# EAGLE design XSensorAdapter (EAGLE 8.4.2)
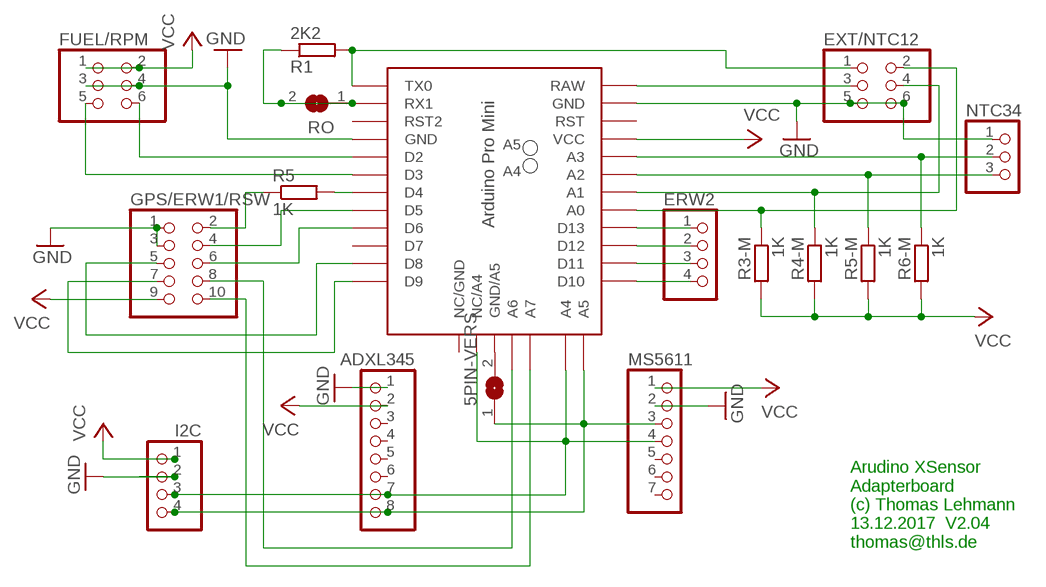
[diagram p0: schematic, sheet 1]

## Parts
5PIN-VERS  SJ  [SJ]
ADXL345  PINHD-1X8  [1X08]
ERW2  PINHD-1X4  [1X04]
EXT/NTC12  PINHD-2X3  [2X03]
FUEL/RPM  PINHD-2X3  [2X03]
GPS/ERW1/RSW  PINHD-2X5  [2X05]
I2C  PINHD-1X4  [1X04]
MS5611  PINHD-1X7  [1X07]
NTC34  PINHD-1X3  [1X03]
R1  2K2  R-EU_0207/10  [0207/10]
R3-M  1K  R-EU_0207/10  [0207/10]
R4-M  1K  R-EU_0207/10  [0207/10]
R5  1K  R-EU_0207/10  [0207/10]
R5-M  1K  R-EU_0207/10  [0207/10]
R6-M  1K  R-EU_0207/10  [0207/10]
RO  SJ  [SJ]
U$1  PRO-MINI-5PINPRO-MINI-5PIN  [PRO-MINI-5PIN]

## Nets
GND: ADXL345.1 EXT/NTC12.5 EXT/NTC12.6 FUEL/RPM.3 FUEL/RPM.4 GPS/ERW1/RSW.1 GPS/ERW1/RSW.3 I2C.2 MS5611.2 NTC34.1 U$1.GND U$1.GND1(GND)
N$1: NTC34.2 R6-M.1 U$1.A3
N$2: EXT/NTC12.1 R1.2 U$1.TX0
N$3: GPS/ERW1/RSW.7 U$1.D9
N$4: EXT/NTC12.3 U$1.RAW
N$5: GPS/ERW1/RSW.10 U$1.A7
N$6: GPS/ERW1/RSW.4 U$1.D5
N$7: GPS/ERW1/RSW.5 U$1.D8
N$8: GPS/ERW1/RSW.6 U$1.D6
N$9: 5PIN-VERS.2 U$1.GND/A5
N$10: EXT/NTC12.2 R3-M.1 U$1.A0
N$11: FUEL/RPM.6 U$1.D2
N$12: R5.2 U$1.D4
N$13: ADXL345.7 I2C.3 MS5611.4 U$1.A5(A4) U$1.NC/A4
N$14: FUEL/RPM.5 U$1.D3
N$15: GPS/ERW1/RSW.2 R5.1
N$16: 5PIN-VERS.1 ADXL345.8 I2C.4 MS5611.3 U$1.A4(A5)
N$17: R1.1 RO.1 RO.2 U$1.RX1
N$18: GPS/ERW1/RSW.8 U$1.A6
N$19: EXT/NTC12.4 R4-M.1 U$1.A1
N$20: NTC34.3 R5-M.1 U$1.A2
N$21: ERW2.1 U$1.D13
N$22: ERW2.2 U$1.D12
N$23: ERW2.3 U$1.D11
N$24: ERW2.4 U$1.D10
VCC: ADXL345.2 FUEL/RPM.1 FUEL/RPM.2 GPS/ERW1/RSW.9 I2C.1 MS5611.1 R3-M.2 R4-M.2 R5-M.2 R6-M.2 U$1.VCC
Unconnected: ADXL345.3 ADXL345.4 ADXL345.5 ADXL345.6 MS5611.5 MS5611.6 MS5611.7 U$1.D7 U$1.NC/GND U$1.RST U$1.RST1(RST2)

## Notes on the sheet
- Arudino XSensor
  Adapterboard
  (c) Thomas Lehmann
  13.12.2017  V2.04
  thomas@thls.de

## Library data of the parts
5PIN-VERS RO = jumper:SJ: SMD solder JUMPER
ADXL345 = pinhead:PINHD-1X8: PIN HEADER
ERW2 I2C = pinhead:PINHD-1X4: PIN HEADER
EXT/NTC12 FUEL/RPM = pinhead:PINHD-2X3: PIN HEADER
GPS/ERW1/RSW = pinhead:PINHD-2X5: PIN HEADER
MS5611 = pinhead:PINHD-1X7: PIN HEADER
NTC34 = pinhead:PINHD-1X3: PIN HEADER
R1 R3-M R4-M R5 R5-M R6-M = resistor:R-EU_: RESISTOR, European symbol
U$1 = OwnLib:PRO-MINI-5PIN

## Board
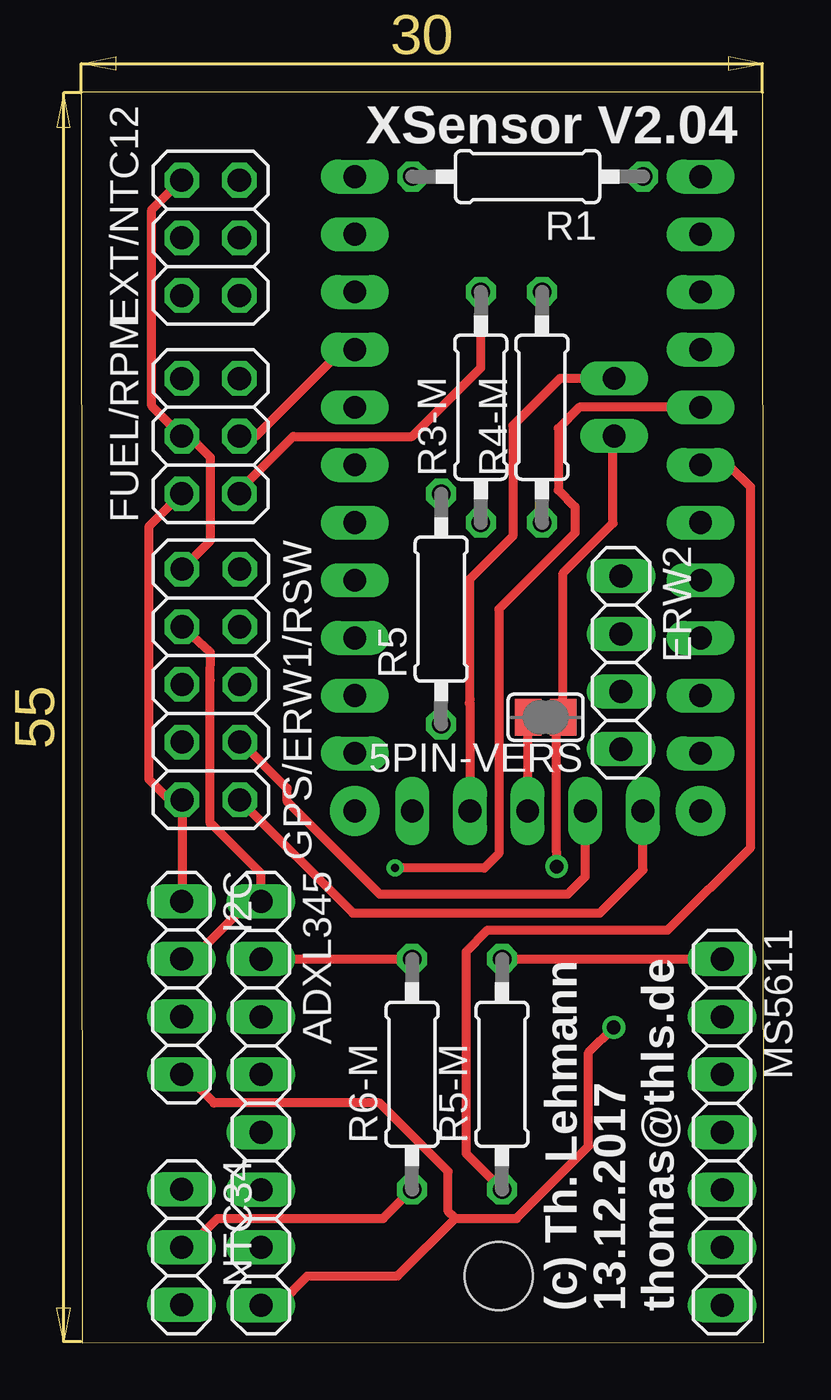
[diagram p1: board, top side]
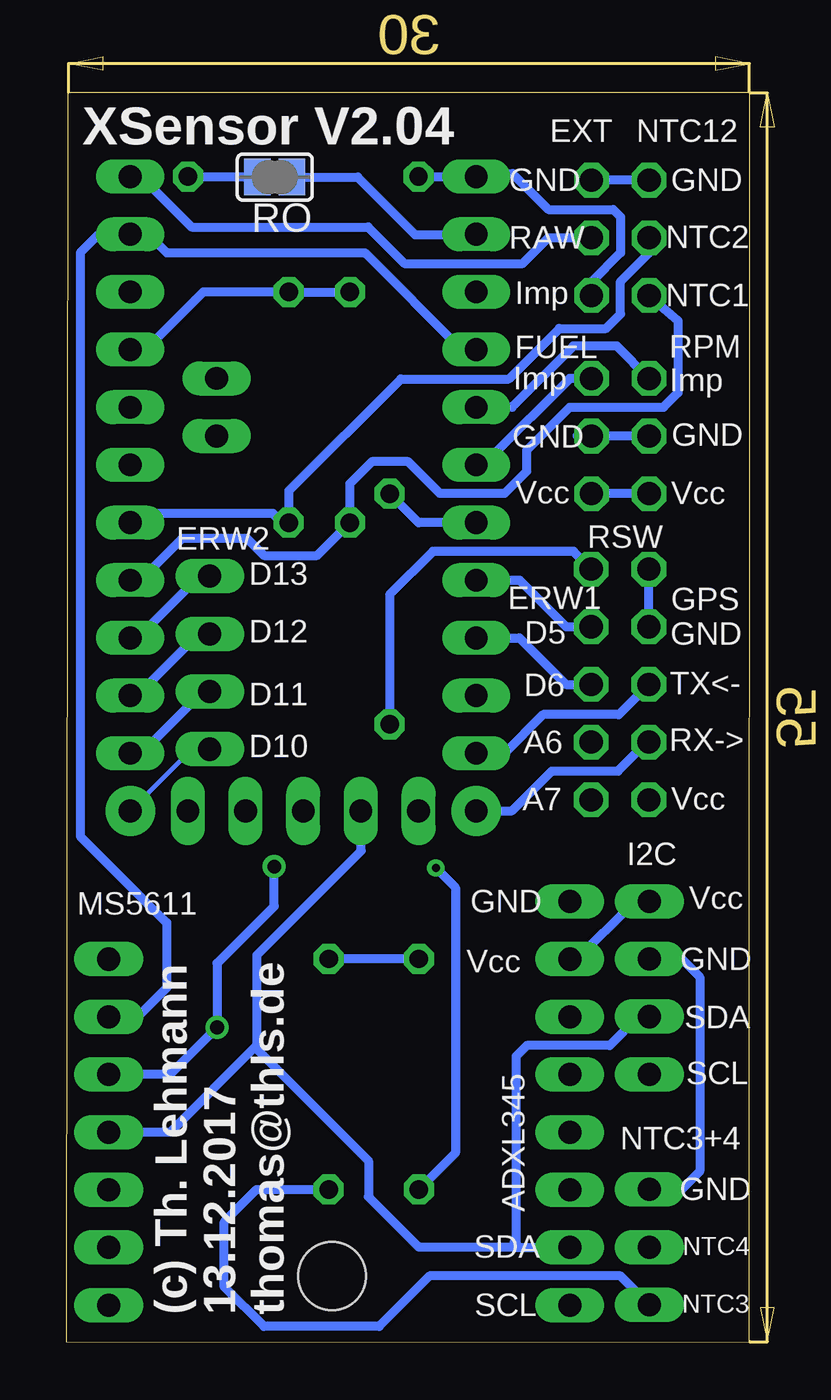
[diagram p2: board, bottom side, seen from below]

Size 31.16 x 56.64 mm. Coordinates in mm from the lower left corner, seen from the top.
Outline: 1.11,0 31.16,0.03 31.11,55.08 1.09,55.08 1.11,0
Copper layers (1*16): Top 0.035mm / dielectric 1.5mm / Bottom 0.035mm
Design rules "Platinenbelichter *": minimum track width 0.2mm, minimum drill 0.6mm, track to track 0.2mm, track to pad 0.2mm, pad to pad 0.2mm, via to via 0.2mm, smd to smd 6mil, copper to edge 0.2mm, drill to drill 0.2mm, minimum pad ring 10mil, minimum via ring 8mil, stop-mask expansion 4mil, vias tented up to drill 0mil, thermal gap 10mil
Holes 3 mm at 19.48,2.95

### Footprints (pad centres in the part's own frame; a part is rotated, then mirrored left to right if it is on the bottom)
SJ = smd 1.168 x 1.6: 1 -0.762,0; 2 0.762,0
1X08 = drill 1.016 long: 1 -8.89,0; 2 -6.35,0; 3 -3.81,0; 4 -1.27,0; 5 1.27,0; 6 3.81,0; 7 6.35,0; 8 8.89,0
1X04 = drill 1.016 long: 1 -3.81,0; 2 -1.27,0; 3 1.27,0; 4 3.81,0
2X03 = drill 1.016 octagon: 1 -2.54,-1.27; 2 -2.54,1.27; 3 0,-1.27; 4 0,1.27; 5 2.54,-1.27; 6 2.54,1.27
2X05 = drill 1.016 octagon: 1 -5.08,-1.27; 2 -5.08,1.27; 3 -2.54,-1.27; 4 -2.54,1.27; 5 0,-1.27; 6 0,1.27; 7 2.54,-1.27; 8 2.54,1.27; 9 5.08,-1.27; 10 5.08,1.27
1X07 = drill 1.016 long: 1 -7.62,0; 2 -5.08,0; 3 -2.54,0; 4 0,0; 5 2.54,0; 6 5.08,0; 7 7.62,0
1X03 = drill 1.016 long: 1 -2.54,0; 2 0,0; 3 2.54,0
0207/10 = drill 0.813 octagon: 1 -5.08,0; 2 5.08,0
PRO-MINI-5PIN = drill 1 long: A0 8.89,8.89; A1 8.89,11.43; A2 8.89,13.97; A3 8.89,16.51; A4 5.08,15.24; A5 5.08,17.78; A6 3.81,-1.27; A7 6.35,-1.27; D2 -6.35,16.51; D3 -6.35,13.97; D4 -6.35,11.43; D5 -6.35,8.89; D6 -6.35,6.35; D7 -6.35,3.81; D8 -6.35,1.27; D11 8.89,1.27; D12 8.89,3.81; D13 8.89,6.35; GND 8.89,24.13; GND1 -6.35,19.05; GND/A5 1.27,-1.27; NC/A4 -1.27,-1.27; NC/GND -3.81,-1.27; RAW 8.89,26.67; RST 8.89,21.59; RST1 -6.35,21.59; RX1 -6.35,24.13; TX0 -6.35,26.67; VCC 8.89,19.05 | drill 1 pad 2.184: D9 -6.35,-1.27; D10 8.89,-1.27

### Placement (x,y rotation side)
5PIN-VERS  21.54,27.55 180 top
ADXL345  9,10.55 270 top
ERW2  24.86,29.95 270 top
EXT/NTC12  6.78,48.67 90 top
FUEL/RPM  6.78,39.94 90 top
GPS/ERW1/RSW  6.79,29 270 top
I2C  5.5,15.64 270 top
MS5611  29.32,9.28 270 top
NTC34  5.5,4.21 270 top
R1  20.75,51.37 180 top
R3-M  18.68,41.21 90 top
R4-M  21.38,41.21 90 top
R5  16.94,32.32 90 top
R5-M  19.62,11.83 90 top
R6-M  15.65,11.83 90 top
RO  22,51.34 180 bottom
U$1  19.48,24.7 0 top

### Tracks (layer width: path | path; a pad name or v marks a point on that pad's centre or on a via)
GND
  Top 0.406: 7.89,39.94 FUEL/RPM.3 8.79,39.94 12.31,43.46 12.31,43.56 12.48,43.73 13.11,43.73 U$1.GND1 | ADXL345.1 8.69,19.13 8.19,19.13 5.97,16.91 I2C.2 | GPS/ERW1/RSW.3 6.78,30.41 6.77,29.18 6.77,22.87 6.8,22.87 9,20.67 ADXL345.1 | ADXL345.1 9,20.1 | GPS/ERW1/RSW.1 6.78,35.33 6.78,39 5.84,39.94 FUEL/RPM.4 4.19,41.26 4.19,49.92 5.47,51.21 EXT/NTC12.6
  Bottom 0.406: FUEL/RPM.4 FUEL/RPM.3 8.68,39.94 | EXT/NTC12.6 EXT/NTC12.5 | U$1.GND1 13.77,43.75 18.03,48.01 26.76,48.01 27.56,48.8 28.34,48.8 U$1.GND 28.39,48.8 29.78,48.8 30.57,48.01 30.57,22.3 26.76,18.49 26.76,15.64 28.04,14.36 MS5611.2 29.33,14.37 | I2C.2 | I2C.2 4.07,16.91 3.27,16.11 3.27,7.54 4.07,6.75 NTC34.1 | GPS/ERW1/RSW.3 GPS/ERW1/RSW.1
N$1  (via drill 0.35)
  Top 0.406: NTC34.2 5.81,4.21 7.08,5.48 14.38,5.48 R6-M.1 | 28.22,41.21 U$1.A3 23.03,41.21 22.09,40.27 22.09,37.55 22.83,36.81 22.83,35.67 19.48,32.32 19.48,21.55 18.84,20.91 v14.9,20.91
  Bottom 0.406: v14.9,20.91 14.04,20.05 14.04,8.36 R6-M.1
N$2
  Bottom 0.406: R1.2 U$1.TX0 12.14,51.37 12,51.5 11.53,51.5 9.94,49.91 7.08,49.91 6.77,49.6 6.77,48.01 8.03,46.74 8.03,46.14 EXT/NTC12.1
N$3
  Bottom 0.406: U$1.D9 11.55,23.43 9.8,25.18 6.88,25.18 5.6,26.46 GPS/ERW1/RSW.7
N$4
  Bottom 0.406: U$1.RAW 27.89,51.37 25.67,49.14 17.89,49.14 16.28,47.53 11.08,47.53 9.95,48.67 EXT/NTC12.3
N$5
  Top 0.406: GPS/ERW1/RSW.10 13.05,18.93 23.92,18.93 25.83,20.83 U$1.A7
N$6
  Bottom 0.406: U$1.D5 11.22,33.59 9.17,31.54 GPS/ERW1/RSW.4
N$7
  Bottom 0.406: GPS/ERW1/RSW.5 6.85,27.67 10.18,27.67 11.88,25.97 U$1.D8
N$8
  Bottom 0.406: U$1.D6 11.22,31.05 9.17,29 GPS/ERW1/RSW.6
N$9
  Top 0.406: 5PIN-VERS.2 20.75,27.52 U$1.GND/A5
N$10
  Bottom 0.406: EXT/NTC12.2 4.24,45.02 4.24,41.84 4.87,41.21 9,41.21 10.9,39.3 10.9,38.38 11.87,37.41 14.73,37.41 15.36,38.05 | 15.36,38.05 15.37,38.05 | 15.36,38.05 16.12,38.81 17.72,38.81 18.68,37.84 R3-M.1 20.13,34.68 22.47,34.68 23.24,35.44 26.06,35.44 27.91,33.59 U$1.A0
N$11
  Bottom 0.406: FUEL/RPM.6 6.93,43.9 8.84,43.9 11.54,41.21 U$1.D2
N$12
  Bottom 0.406: U$1.D4 15.67,36.13 R5.2
N$13
  Top 0.406: U$1.A5 22.18,42.48 20.1,40.39 20.1,35.53 18.18,33.61 18.18,28.18 18.21,28.15 | 18.21,28.15 18.21,28.35 | 18.21,28.15 U$1.NC/A4
  Bottom 0.406: 22.79,13.1 22.79,17.06 18.19,21.67 18.19,23.41 U$1.NC/A4 | 22.79,13.1 22.79,12.94 17.87,8.02 17.87,6.43 15.65,4.21 11.37,4.21 | 11.37,4.21 11.21,4.21 | 11.21,4.21 9.01,4.21 ADXL345.7 | 11.44,4.44 11.21,4.21 | I2C.3 5.97,14.37 7.24,13.1 10.89,13.1 11.37,12.62 11.37,4.21 | 22.79,13.1 26.61,9.28 MS5611.4
N$14
  Bottom 0.406: FUEL/RPM.5 9,42.48 12.49,38.98 U$1.D3
N$15
  Bottom 0.406: GPS/ERW1/RSW.2 8.84,34.86 15.03,34.86 16.94,32.95 R5.1
N$16  (via drill 0.6)
  Top 0.406: 22.32,27.57 5PIN-VERS.1 | 5PIN-VERS.1 22.63,27.22 | 9.01,1.67 ADXL345.8 9.77,1.66 11.05,2.94 15.02,2.94 17.56,5.48 | 17.56,5.48 20.25,5.48 23.43,8.65 23.43,12.78 v24.54,13.89 | 17.56,5.48 17.24,5.8 17.24,7.54 14.22,10.56 6.92,10.56 5.66,11.83 I2C.4 | 5PIN-VERS.1 22.02,27.27 22.02,21.6 22.03,21.59 v22.03,20.98 | 5PIN-VERS.1 22.3,33.9 24.51,36.1 24.51,39.88 U$1.A4
  Bottom 0.406: v22.03,20.98 22.03,19.23 24.54,16.71 v24.54,13.89 26.61,11.82 MS5611.3
N$17
  Bottom 0.406: U$1.RX1 13.15,48.8 15.81,48.8 18.35,51.34 RO.1 RO.2 22.78,51.37 R1.1
N$18
  Top 0.406: GPS/ERW1/RSW.8 8.11,26.46 10.15,24.42 10.15,23.83 14.22,19.76 22.52,19.76 23.29,20.53 U$1.A6
N$19
  Bottom 0.406: EXT/NTC12.4 5.51,48 6.77,46.74 6.77,45.31 7.4,44.68 9.46,44.68 11.68,42.46 16.45,42.46 21.38,37.52 R4-M.1 21.69,36.13 22.09,36.53 27.96,36.53 U$1.A1 | U$1.A1
N$20
  Top 0.406: R5-M.1 18.03,8.33 18.03,17.22 18.99,18.17 26.92,18.17 30.57,21.82 30.57,37.69 29.62,38.65 28.38,38.65 U$1.A2
  Bottom 0.406: NTC34.3 6.77,2.94 15.18,2.94 17.4,0.72 22.48,0.72 24.22,2.46 24.22,5.32 22.8,6.75 R5-M.1
N$21
  Bottom 0.406: U$1.D13 28.04,31.05 25.39,33.69 24.94,33.69 ERW2.1
N$22
  Bottom 0.406: U$1.D12 28.06,28.51 25.47,31.1 24.99,31.1 ERW2.2
N$23
  Bottom 0.406: U$1.D11 27.88,25.97 25.24,28.61 ERW2.3
N$24
  Bottom 0.203: U$1.D10 25.72,26.07
  Bottom 0.406: 25.72,26.07 ERW2.4
VCC
  Top 0.406: FUEL/RPM.1 8.05,37.55 10.42,39.92 15.65,39.92 18.68,42.95 R3-M.2 | ADXL345.2 15.64,16.9 R6-M.2 | R5-M.2 29.31,16.91 MS5611.1 | I2C.1 5.52,19.47 GPS/ERW1/RSW.9 4.96,23.92 4.06,24.82 4.06,35.95 FUEL/RPM.2
  Bottom 0.406: FUEL/RPM.2 FUEL/RPM.1 | R3-M.2 R4-M.2 25.15,46.29 27.69,43.75 U$1.VCC | ADXL345.2 8.68,16.9 6.29,19.29 5.66,19.29 I2C.1 | 15.64,16.9 R6-M.2 R5-M.2

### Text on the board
tNames: XSensor V2.04 | (c) Th. Lehmann / 13.12.2017 / thomas@thls.de
bNames: XSensor V2.04 | NTC12 | EXT | GND | GND | NTC2 | RAW | Imp | NTC1 | RPM | FUEL | Imp | Imp | GND | GND | Vcc | Vcc | RSW | ERW2 | D13 | GPS | ERW1 | D5 | D12 | GND | TX<- | D6 | D11 | RX-> | A6 | D10 | Vcc | A7 | I2C | Vcc | GND | MS5611 | GND | Vcc | SDA | ADXL345 | SCL | NTC3+4 | GND | NTC4 | SDA | NTC3 | SCL | (c) Th. Lehmann / 13.12.2017 / thomas@thls.de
